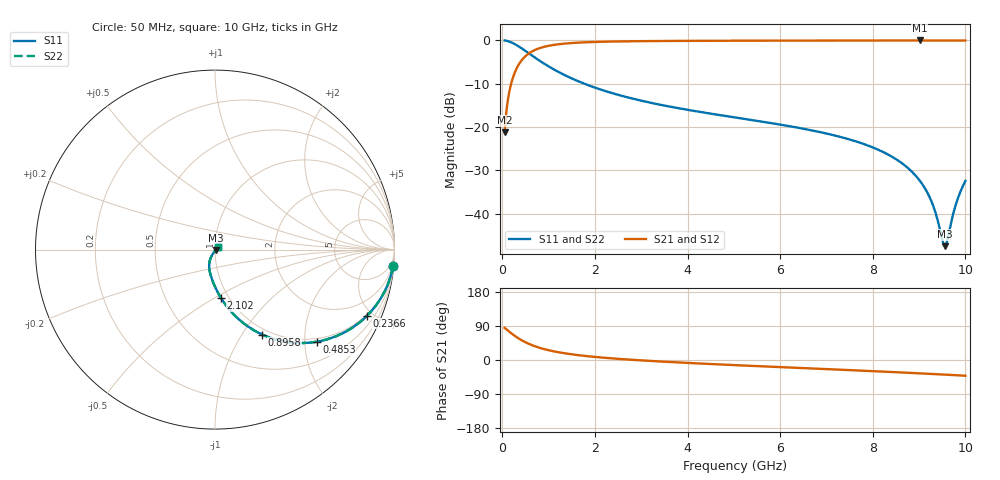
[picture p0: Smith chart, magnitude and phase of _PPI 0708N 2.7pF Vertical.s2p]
! S-Parameter data specifications (vertical orientation):
! Substrate: 40-mil Rogers 3003C, Substrate thickness, H=1.016mm, Dielectric constant, Er=3, Conductor thickness, T_mtl=0.043mm, Loss Tangent, Tand=0.003
! PCB Mounting Pad Footprint: Pad width, PadW=2.54mm , Pad length, PadL=0.51mm , Pad gap, PadG (edge-to-edge)=0.71mm , Reference planes=1.73mm apart
! Created Tue Jan 16 08:44:43 2018
# GHz S MA R 50
! 2 Port Network Data from SP1.SP block
! freq  magS11  angS11  magS21  angS21  magS12  angS12  magS22  angS22
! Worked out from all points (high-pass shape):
!   801 points, 50 MHz to 10 GHz, reference 50 ohm
!   highest |S21| = -0.04 dB at 9.017 GHz (marker M1); lowest = -21.2 dB at 50 MHz (marker M2)
!   |S21| within 3 dB of the highest: 572.4 MHz to end of sweep
!   lowest |S11| = -47.4 dB at 9.552 GHz (marker M3), VSWR 1.01, Z = 50.3 - j0.29 ohm
!   |S11| at or under -10 dB: 1.772 GHz to end of sweep
!   |S22| runs from -47.4 to 0.0 dB; largest |S21 - S12| = 0
!   S11 on the Smith chart (normalised r, x): 50 MHz: 1, -22; 236.6 MHz: 0.92, -4.65; 485.3 MHz: 0.92, -2.27; 895.8 MHz: 0.92, -1.24; 2.102 GHz: 0.92, -0.54; 10 GHz: 1.04, +0.03
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0.05  0.9962 -5.2  0.08684 84.8  0.08684 84.8  0.9962 -5.2
0.1495  0.9676 -15.2  0.2521 74.8  0.2521 74.8  0.9676 -15.2
0.2365625  0.9245 -23.4  0.381 66.6  0.381 66.6  0.9245 -23.4
0.3485  0.8548 -32.7  0.5187 57.3  0.5187 57.3  0.8548 -32.7
0.4853125  0.764 -42.2  0.6448 47.8  0.6448 47.8  0.764 -42.2
0.89575  0.5421 -60.9  0.8396 29.0  0.8396 29.0  0.5421 -60.9
1.244  0.4238 -70.1  0.9049 19.8  0.9049 19.8  0.4238 -70.1
1.716625  0.3248 -78.1  0.9447 11.7  0.9447 11.7  0.3248 -78.1
2.102187  0.2732 -82.8  0.9608 7.0  0.9608 7.0  0.2732 -82.8
3.370812  0.1828 -93.2  0.9816 -3.7  0.9816 -3.7  0.1828 -93.2
5.025  0.1292 -102.7  0.9896 -13.6  0.9896 -13.6  0.1292 -102.7
6.691625  0.09152 -110.9  0.9932 -22.4  0.9932 -22.4  0.09152 -110.9
7.649312  0.06809 -115.1  0.9946 -27.5  0.9946 -27.5  0.06809 -115.1
8.345812  0.04779 -117.5  0.9954 -31.3  0.9954 -31.3  0.04779 -117.5
8.731375  0.03475 -117.8  0.9956 -33.5  0.9956 -33.5  0.03475 -117.8
9.017437  0.02404 -116.4  0.9957 -35.2  0.9957 -35.2  0.02404 -116.4
9.278625  0.01347 -109.9  0.9956 -36.8  0.9956 -36.8  0.01347 -109.9
9.5025  0.00497 -71.1  0.9954 -38.2  0.9954 -38.2  0.00497 -71.1
9.55225  0.004247 -42.7  0.9954 -38.5  0.9954 -38.5  0.004247 -42.7
9.602  0.004794 -12.5  0.9953 -38.9  0.9953 -38.9  0.004794 -12.5
9.825875  0.01446 31.1  0.9949 -40.4  0.9949 -40.4  0.01446 31.1
10  0.02401 36.8  0.9945 -41.6  0.9945 -41.6  0.02401 36.8
